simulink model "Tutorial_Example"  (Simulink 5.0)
settings: Solver=FixedStepDiscrete  StartTime=0  StopTime=5356800  FixedStep=300  RelTol=1e-3
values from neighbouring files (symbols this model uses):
  table = A(2:end,1:end)    [CD1_mfun_rainread.m]    (also in CD1_sfun_rainread.m = [table; table(end,1)+tablestep -1])
  tablestep = tableEnd-tableStart    [CD1_sfun_flowread.m]

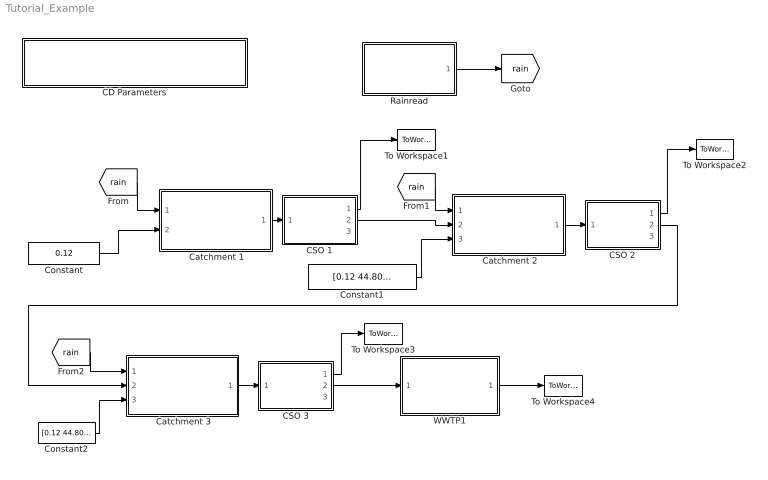
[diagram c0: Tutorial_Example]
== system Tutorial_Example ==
  " Catchment 1" : Subsystem  mask(Catchment CSS - Type A){area=200, rfcoeff=1, initloss=1, permloss=2, n_ta=5, n_comp=3, Rain_C=[5.7 0.65 3], DWF_C=[44.80 13.89 18.00]}
      mask prompts: area "Area in [ha]"; rfcoeff "Runoff coefficient (0 - 1)"; initloss "Initial Loss in [mm]"; permloss "Permanent loss in [mm/day]"; n_ta "No of Timesteps (transport time) / No of subareas n [-]"; n_comp "No of pollutant components"; Rain_C "Vector of Rain-Conc. [g/m3]"; DWF_C "Vector of DWF-Conc. [g/m3]"
      mask help: Simple model of an urban catchment with Combined sewer system (CSS). Input ( r ) is a continuous stream of rain data in [mm/DT]. Input (dwf) is the dry weather flow in [m3/s]. Pollutants concentrations are considered as constant over time. The block contains an initial loss model for runoff generation, a time-area model for overland flow computation and a mixing model for computing runoff concentrations for n components.
      mask init:
      | % location of catchment drawing
      | x=0;
      | y=-10;
      | % reading the toplevel systems' name 
      | % --> Plant file name;
      | tls=bdroot(gcb); 
      | % Obtaining the fixed sampling time
      | t_samp_char=get_param(tls, 'FixedStep');
      | % Convertion to numeric value
      | tstep = str2num(t_samp_char); 
      | 
      | %convertion form mm/day --> mm/DT
      | permloss=permloss/86400*tstep;
      | 
      | area=area.*10000;
  " Catchment 2" : Subsystem  mask(Catchment CSS - Type B){area=200, rfcoeff=1, initloss=1, permloss=2, n_ta=5, n_comp=3, Rain_C=[5.7 0.65 3]}
      mask prompts: area "Area in [ha]"; rfcoeff "Runoff coefficient (0 - 1)"; initloss "Initial Loss in [mm]"; permloss "Permanent loss in [mm/day]"; n_ta "No of Timesteps (transport time) / No of subareas n [-]"; n_comp "No of pollutant components"; Rain_C "Vector of Rain-Conc. [g/m3]"
      mask help: Simple model of an urban catchment. Input ( r ) is a continuous stream of rain data in [mm/DT]. Input (DWF) is the dry weather flow. Input (QP) is the parasite water flow entering. Pollutants concentrations for rain are considered constant over time. The block contains an initial loss model for runoff generation, a time/area model for overland flow computation and a mixing model for computing runoff concentrations for n components.
      mask init:
      | % location of catchment drawing
      | x=0;
      | y=-10;
      | % reading the toplevel systems' name 
      | % --> Plant file name;
      | tls=bdroot(gcb); 
      | % Obtaining the fixed sampling time
      | t_samp_char=get_param(tls, 'FixedStep');
      | % Convertion to numeric value
      | tstep = str2num(t_samp_char); 
      | 
      | %convertion form mm/day --> mm/DT
      | permloss=permloss/86400*tstep;
      | 
      | area=area.*10000;
  " Catchment 3" : Subsystem  mask(Catchment CSS - Type B){area=200, rfcoeff=1, initloss=1, permloss=2, n_ta=5, n_comp=3, Rain_C=[5.7 0.65 3]}
      mask prompts: area "Area in [ha]"; rfcoeff "Runoff coefficient (0 - 1)"; initloss "Initial Loss in [mm]"; permloss "Permanent loss in [mm/day]"; n_ta "No of Timesteps (transport time) / No of subareas n [-]"; n_comp "No of pollutant components"; Rain_C "Vector of Rain-Conc. [g/m3]"
      mask help: Simple model of an urban catchment. Input ( r ) is a continuous stream of rain data in [mm/DT]. Input (DWF) is the dry weather flow. Input (QP) is the parasite water flow entering. Pollutants concentrations for rain are considered constant over time. The block contains an initial loss model for runoff generation, a time/area model for overland flow computation and a mixing model for computing runoff concentrations for n components.
      mask init:
      | % location of catchment drawing
      | x=0;
      | y=-10;
      | % reading the toplevel systems' name 
      | % --> Plant file name;
      | tls=bdroot(gcb); 
      | % Obtaining the fixed sampling time
      | t_samp_char=get_param(tls, 'FixedStep');
      | % Convertion to numeric value
      | tstep = str2num(t_samp_char); 
      | 
      | %convertion form mm/day --> mm/DT
      | permloss=permloss/86400*tstep;
      | 
      | area=area.*10000;
  CD Parameters : Subsystem  mask(City Drain 1.0 - Simulation parameters ){t_step=300, t_start=0, t_stop=2*2678400}
      mask prompts: t_step "Sampling Time [s]"; t_start "Start Time [s]"; t_stop "Stop Time [s]"
      mask help: Block that sets the global parameters required in City Drain 1.0. Following paramters are set without user's input: - 'Solver' --> 'FixedStepDiscrete' - 'TimeSaveName' --> 'cd_time' - 'Decimation' --> '1' - 'LimitDataPoints' --> 'off'
      mask init:
      | % toplevel systems' name --> Plant file name;
      | tls=bdroot(gcb); 
      | set_param(tls, 'Solver', 'FixedStepDiscrete'); 
      | set_param(tls, 'TimeSaveName', 'cd_time');
      | set_param(tls, 'Decimation', '1');
      | set_param(tls, 'LimitDataPoints', 'off');
      | set_param(tls, 'ScreenColor', 'white');
      | 
      | tstep_char=num2str(t_step); % Setting the discrete time step
      | set_param(tls, 'FixedStep', tstep_char); 
      | 
      | tstart_char=num2str(t_start); % Setting the start time
      | set_param(tls, 'StartTime', tstart_char); 
      | 
      | tstop_char=num2str(t_stop); % Setting the stop time
      | set_param(tls, 'StopTime', tstop_char);
  CSO 1 : Subsystem  mask(CSO Typ A - Combined sewer overflow){Vmax=3000, Qemax=0.52, n_comp=3}
      mask prompts: Vmax "Basin Volume [m3]"; Qemax "Maximum Effluent flow [m3/s]"; n_comp "Number of Pollutants [-]"
      mask help: Combined sewer overflow structure. Diverts the inflow given into effluent and overflow. The model implemented consideres hydraulics and pollutant routing by full mixing in the structure. Function used: CD1_sfun_cso_A.m
      mask init:
      | % reading the toplevel systems' name 
      | % --> Plant file name;
      | tls=bdroot(gcb); 
      | % Obtaining the fixed sampling time
      | t_samp_char=get_param(tls, 'FixedStep');
      | % Convertion to numeric value
      | tstep = str2num(t_samp_char);
  CSO 2 : Subsystem  mask(CSO Typ A - Combined sewer overflow){Vmax=3775, Qemax=1.04, n_comp=3}
      mask prompts: Vmax "Basin Volume [m3]"; Qemax "Maximum Effluent flow [m3/s]"; n_comp "Number of Pollutants [-]"
      mask help: Combined sewer overflow structure. Diverts the inflow given into effluent and overflow. The model implemented consideres hydraulics and pollutant routing by full mixing in the structure. Function used: CD1_sfun_cso_A.m
      mask init:
      | % reading the toplevel systems' name 
      | % --> Plant file name;
      | tls=bdroot(gcb); 
      | % Obtaining the fixed sampling time
      | t_samp_char=get_param(tls, 'FixedStep');
      | % Convertion to numeric value
      | tstep = str2num(t_samp_char);
  CSO 3 : Subsystem  mask(CSO Typ A - Combined sewer overflow){Vmax=4870, Qemax=1.56, n_comp=3}
      mask prompts: Vmax "Basin Volume [m3]"; Qemax "Maximum Effluent flow [m3/s]"; n_comp "Number of Pollutants [-]"
      mask help: Combined sewer overflow structure. Diverts the inflow given into effluent and overflow. The model implemented consideres hydraulics and pollutant routing by full mixing in the structure. Function used: CD1_sfun_cso_A.m
      mask init:
      | % reading the toplevel systems' name 
      | % --> Plant file name;
      | tls=bdroot(gcb); 
      | % Obtaining the fixed sampling time
      | t_samp_char=get_param(tls, 'FixedStep');
      | % Convertion to numeric value
      | tstep = str2num(t_samp_char);
  Constant : Constant  Value=0.12
  Constant1 : Constant  Value=[0.12 44.80 13.89 18.00]
  Constant2 : Constant  Value=[0.12 44.80 13.89 18.00]
  Rainread : Subsystem  mask(Rain Read){table0='Input_ixx_1y_example.ixx', crep=off}
      mask prompts: table0 "Filename"; crep "Cylic repitition"
      mask help: Read raindata from ASCII File in following formats: *.ixx ... Format used by the Austrian Hydrographic Service. *.km2 ... Format used in the Mouse Software from DHI (Danish Hydraulic Institute) *.mse ... modified mse format used in Mouse Software from DHI (Danish Hydraulic Institute) Used function: CD1_mfun_rainread.m
      mask init:
      | % cache table size set to 1000
      | %table=zeros(1000,2)
      | [table,tablestep]=CD1_mfun_rainread(table0);
      | 
      | % reading the toplevel systems' name 
      | % --> Plant file name;
      | tls=bdroot(gcb); 
      | % Obtaining the fixed sampling time
      | t_samp_char=get_param(tls, 'FixedStep');
      | % Convertion to numeric value
      | tstep = str2num(t_samp_char);
  To Workspace1 : ToWorkspace  VariableName=Qw1  SampleTime=-1  SaveFormat=Array
  To Workspace2 : ToWorkspace  VariableName=Qw2  SampleTime=-1  SaveFormat=Array
  To Workspace3 : ToWorkspace  VariableName=Qw3  SampleTime=-1  SaveFormat=Array
  To Workspace4 : ToWorkspace  VariableName=Qw  SampleTime=-1  SaveFormat=Array
  WWTP1 : Subsystem  mask(WWTP){REmin=[0.8  0.9 0.9], Cemax=[100 100 100], n_comp=3}
      mask prompts: REmin "Removal Efficiency REmin [-]"; Cemax "Maximum effluent concnetration Cemax [g/m³]"; n_comp "Number of Components ()"
      mask help: Simple WWTP model. Inflow given is treated according to userdefined maximum concnetration limits and treatment efficiencies. Function used: CD1_sfun_WWTP.m
      mask init:
      | % reading the toplevel systems' name 
      | % --> Plant file name;
      | tls=bdroot(gcb); 
      | % Obtaining the fixed sampling time
      | t_samp_char=get_param(tls, 'FixedStep');
      | % Convertion to numeric value
      | tstep = str2num(t_samp_char); 
      | 
      | RE=REmin;
      | for i=1:n_comp
      | 	if REmin(i) < 0 
      | 		RE(i)=0;
      | 		fprintf('WARNING, Block WWTP:  Removal efficientc of component %u has set to 0, User input REmin <0 \n',i);
      | 	elseif REmin(i) > 1
      | 		RE(i)=1;
      | 		fprintf('WARNING, Block WWTP:  Removal efficientc of component %u has set to 1, User input REmin >1 \n',i);
      | 	else
      | 		RE(i)=REmin(i);
      | 	end
      | end
      | fprintf('\n');
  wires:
  Rainread/1(out_1) -> [rain]
  " Catchment 1"/1(Runoff vector Q,C) -> CSO 1/1(In)
  Constant/1 -> " Catchment 1"/2(DWF(m3/s))
  [rain] -> " Catchment 1"/1(Rain (mm/dt))
  CSO 1/1(Qw) -> To Workspace1/1
  CSO 1/2(Qe) -> " Catchment 2"/2(DWF(m3/s))
  Constant1/1 -> " Catchment 2"/3(QP)
  " Catchment 2"/1(Runoff vector Q,C) -> CSO 2/1(In)
  [rain] -> " Catchment 2"/1(Rain (mm/dt))
  CSO 2/1(Qw) -> To Workspace2/1
  " Catchment 3"/1(Runoff vector Q,C) -> CSO 3/1(In)
  Constant2/1 -> " Catchment 3"/3(QP)
  CSO 3/2(Qe) -> WWTP1/1(In)
  [rain] -> " Catchment 3"/1(Rain (mm/dt))
  CSO 3/1(Qw) -> To Workspace3/1
  WWTP1/1(Qw) -> To Workspace4/1
  CSO 2/2(Qe) -> " Catchment 3"/2(DWF(m3/s))

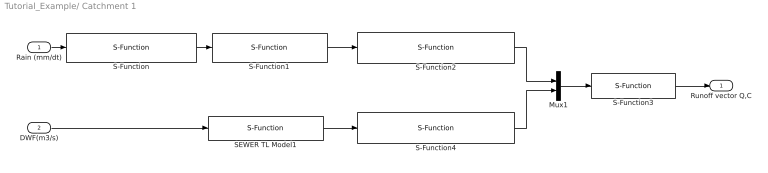
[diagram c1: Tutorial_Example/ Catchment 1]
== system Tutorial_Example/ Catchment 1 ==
  Rain (mm/dt) : Inport
  DWF(m3/s) : Inport  Port=2
  Mux1 : Mux  Inputs=[n_comp+1,n_comp+1]
  S-Function : S-Function  FunctionName=CD1_sfun_catchment_lossmodel  Parameters=initloss,permloss,rfcoeff
  S-Function1 : S-Function  FunctionName=CD1_sfun_catchment_tamodel  Parameters=n_ta
  S-Function2 : S-Function  FunctionName=CD1_sfun_catchment_flowmodel_SW  Parameters=area,n_comp,Rain_C,tstep
  S-Function3 : S-Function  FunctionName=CD1_sfun_mixing_QC  Parameters=n_comp,tstep
  S-Function4 : S-Function  FunctionName=CD1_sfun_catchment_flowmodel_DWF  Parameters=n_comp,DWF_C,tstep
  SEWER TL Model1 : S-Function  FunctionName=CD1_sfun_sewer_tlmodel  Parameters=n_ta,0,tstep
  Runoff vector Q,C : Outport
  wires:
  S-Function4/1 -> Mux1/2
  S-Function2/1 -> Mux1/1
  SEWER TL Model1/1 -> S-Function4/1
  S-Function1/1 -> S-Function2/1
  S-Function3/1 -> Runoff vector Q,C/1
  Mux1/1 -> S-Function3/1
  DWF(m3/s)/1 -> SEWER TL Model1/1
  Rain (mm/dt)/1 -> S-Function/1
  S-Function/1 -> S-Function1/1

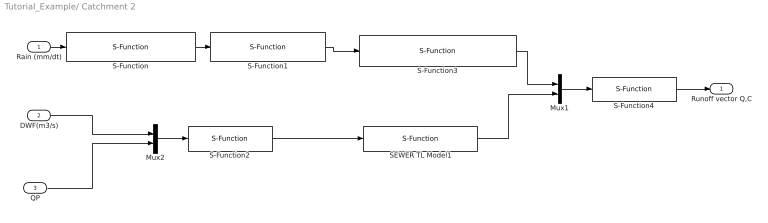
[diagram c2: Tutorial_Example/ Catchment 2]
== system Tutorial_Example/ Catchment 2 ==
  Rain (mm/dt) : Inport
  DWF(m3/s) : Inport  Port=2
  QP : Inport  Port=3
  Mux1 : Mux  Inputs=[n_comp+1,n_comp+1]
  Mux2 : Mux  Inputs=[n_comp+1,n_comp+1]
  S-Function : S-Function  FunctionName=CD1_sfun_catchment_lossmodel  Parameters=initloss,permloss,rfcoeff
  S-Function1 : S-Function  FunctionName=CD1_sfun_catchment_tamodel  Parameters=n_ta
  S-Function2 : S-Function  FunctionName=CD1_sfun_mixing_QC  Parameters=n_comp,tstep
  S-Function3 : S-Function  FunctionName=CD1_sfun_catchment_flowmodel_SW  Parameters=area,n_comp,Rain_C,tstep
  S-Function4 : S-Function  FunctionName=CD1_sfun_mixing_QC  Parameters=n_comp,tstep
  SEWER TL Model1 : S-Function  FunctionName=CD1_sfun_sewer_tlmodel  Parameters=n_ta,n_comp,tstep
  Runoff vector Q,C : Outport
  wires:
  S-Function/1 -> S-Function1/1
  Rain (mm/dt)/1 -> S-Function/1
  Mux1/1 -> S-Function4/1
  S-Function4/1 -> Runoff vector Q,C/1
  S-Function3/1 -> Mux1/1
  S-Function1/1 -> S-Function3/1
  Mux2/1 -> S-Function2/1
  S-Function2/1 -> SEWER TL Model1/1
  DWF(m3/s)/1 -> Mux2/1
  QP/1 -> Mux2/2
  SEWER TL Model1/1 -> Mux1/2

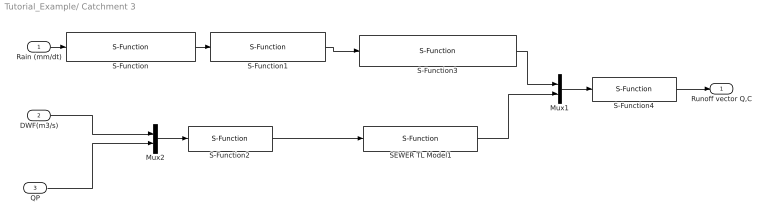
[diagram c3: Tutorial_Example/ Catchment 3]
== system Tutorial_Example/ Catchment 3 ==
  Rain (mm/dt) : Inport
  DWF(m3/s) : Inport  Port=2
  QP : Inport  Port=3
  Mux1 : Mux  Inputs=[n_comp+1,n_comp+1]
  Mux2 : Mux  Inputs=[n_comp+1,n_comp+1]
  S-Function : S-Function  FunctionName=CD1_sfun_catchment_lossmodel  Parameters=initloss,permloss,rfcoeff
  S-Function1 : S-Function  FunctionName=CD1_sfun_catchment_tamodel  Parameters=n_ta
  S-Function2 : S-Function  FunctionName=CD1_sfun_mixing_QC  Parameters=n_comp,tstep
  S-Function3 : S-Function  FunctionName=CD1_sfun_catchment_flowmodel_SW  Parameters=area,n_comp,Rain_C,tstep
  S-Function4 : S-Function  FunctionName=CD1_sfun_mixing_QC  Parameters=n_comp,tstep
  SEWER TL Model1 : S-Function  FunctionName=CD1_sfun_sewer_tlmodel  Parameters=n_ta,n_comp,tstep
  Runoff vector Q,C : Outport
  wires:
  S-Function/1 -> S-Function1/1
  Rain (mm/dt)/1 -> S-Function/1
  Mux1/1 -> S-Function4/1
  S-Function4/1 -> Runoff vector Q,C/1
  S-Function3/1 -> Mux1/1
  S-Function1/1 -> S-Function3/1
  Mux2/1 -> S-Function2/1
  S-Function2/1 -> SEWER TL Model1/1
  DWF(m3/s)/1 -> Mux2/1
  QP/1 -> Mux2/2
  SEWER TL Model1/1 -> Mux1/2

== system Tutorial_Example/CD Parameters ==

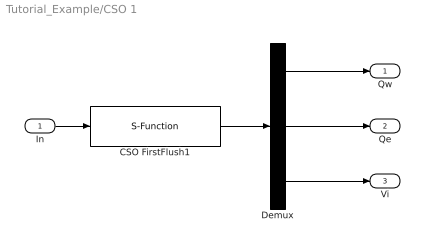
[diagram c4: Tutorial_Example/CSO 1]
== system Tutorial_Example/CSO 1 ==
  In : Inport
  CSO FirstFlush1 : S-Function  FunctionName=CD1_sfun_cso_A  Parameters=Vmax,Qemax,n_comp,tstep
  Demux : Demux  Outputs=[ (n_comp+1) (n_comp+1) (n_comp+1)]
  Qw : Outport
  Qe : Outport  Port=2
  Vi : Outport  Port=3
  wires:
  Demux/3 -> Vi/1
  Demux/2 -> Qe/1
  Demux/1 -> Qw/1
  CSO FirstFlush1/1 -> Demux/1
  In/1 -> CSO FirstFlush1/1

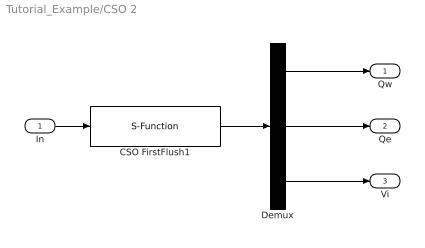
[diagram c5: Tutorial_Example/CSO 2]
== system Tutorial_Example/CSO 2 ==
  In : Inport
  CSO FirstFlush1 : S-Function  FunctionName=CD1_sfun_cso_A  Parameters=Vmax,Qemax,n_comp,tstep
  Demux : Demux  Outputs=[ (n_comp+1) (n_comp+1) (n_comp+1)]
  Qw : Outport
  Qe : Outport  Port=2
  Vi : Outport  Port=3
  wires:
  Demux/3 -> Vi/1
  Demux/2 -> Qe/1
  Demux/1 -> Qw/1
  CSO FirstFlush1/1 -> Demux/1
  In/1 -> CSO FirstFlush1/1

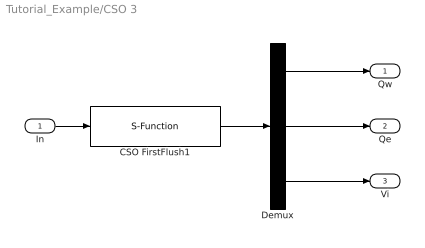
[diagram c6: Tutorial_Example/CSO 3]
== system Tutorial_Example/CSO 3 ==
  In : Inport
  CSO FirstFlush1 : S-Function  FunctionName=CD1_sfun_cso_A  Parameters=Vmax,Qemax,n_comp,tstep
  Demux : Demux  Outputs=[ (n_comp+1) (n_comp+1) (n_comp+1)]
  Qw : Outport
  Qe : Outport  Port=2
  Vi : Outport  Port=3
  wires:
  Demux/3 -> Vi/1
  Demux/2 -> Qe/1
  Demux/1 -> Qw/1
  CSO FirstFlush1/1 -> Demux/1
  In/1 -> CSO FirstFlush1/1

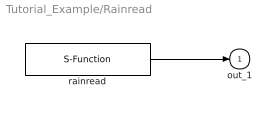
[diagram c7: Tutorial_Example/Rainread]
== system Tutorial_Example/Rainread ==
  rainread : S-Function  FunctionName=CD1_sfun_rainread  Parameters=crep,table,tablestep,tstep
  out_1 : Outport
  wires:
  rainread/1 -> out_1/1

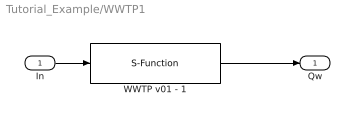
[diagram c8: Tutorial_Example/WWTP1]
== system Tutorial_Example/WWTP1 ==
  In : Inport
  WWTP v01 - 1 : S-Function  FunctionName=CD1_sfun_WWTP  Parameters=n_comp,RE,Cemax,tstep
  Qw : Outport
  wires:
  In/1 -> WWTP v01 - 1/1
  WWTP v01 - 1/1 -> Qw/1
